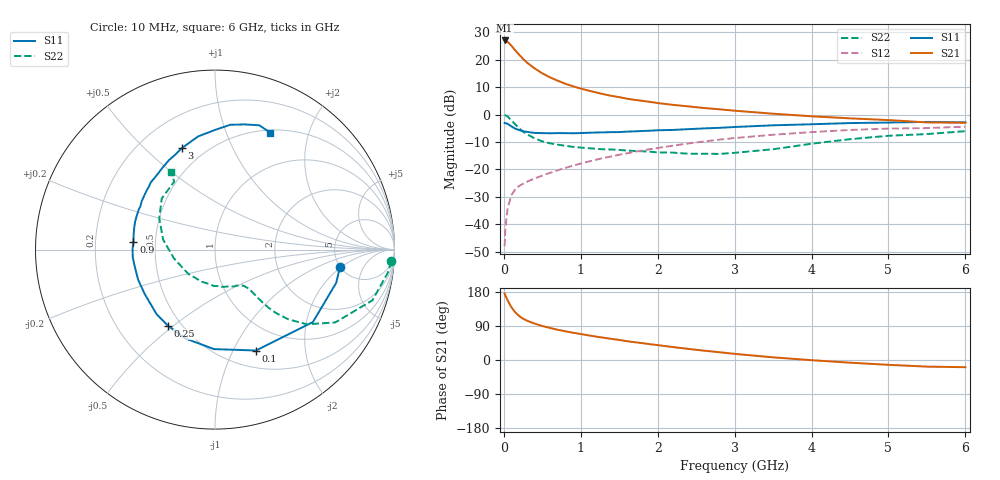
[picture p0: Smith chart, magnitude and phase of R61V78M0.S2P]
! SIEMENS Small Signal Semiconductors
! BFR193
! Si NPN RF Bipolar Junction Transistor in SOT23
! VCE = 1.75 V  IC = 8 mA
! Common Emitter S-Parameters:  May  1996
# GHz  S  MA  R  50
!  f  S11  S21  S12  S22
! GHz  MAG  ANG  MAG  ANG  MAG  ANG  MAG  ANG
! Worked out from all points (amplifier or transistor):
!   36 points, 10 MHz to 6 GHz, reference 50 ohm
!   highest |S21| = 27.0 dB at 10 MHz (marker M1)
!   |S21| within 3 dB of that: start of sweep to 130.2 MHz
!   unconditionally stable (mu >= 1): 771.2 MHz to 1.99 GHz
!   at 250 MHz: K = 0.58, MSG = 22.8 dB, |S12| = -25.2 dB
!   at 1.4 GHz: K = 1.05, MAG = 9.7 dB, |S12| = -15.2 dB
!   at 6 GHz: K = 0.96, MSG = 0.7 dB, |S12| = -4.4 dB
!   S11 on the Smith chart (normalised r, x): 10 MHz: 4.99, -1.88; 100 MHz: 0.69, -1.23; 250 MHz: 0.42, -0.48; 900 MHz: 0.37, +0.04; 3 GHz: 0.37, +0.65; 6 GHz: 0.53, +1.44
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0.01  0.7027 -7.8  22.46 175.3  0.004 88.2  0.9843 -3.8
0.02  0.7004 -15.3  22.03 170.3  0.0085 82.0  0.973 -7.4
0.05  0.6785 -36.5  21.13 157.0  0.0199 72.7  0.9212 -17.9
0.1  0.6068 -67.9  17.96 138.7  0.0345 62.0  0.7833 -31.2
0.15  0.5544 -90.6  14.69 125.3  0.0437 55.9  0.66 -39.1
0.2  0.5219 -108.3  12.32 116.0  0.05 53.0  0.5609 -43.7
0.25  0.4985 -121.7  10.37 109.0  0.055 51.9  0.487 -46.2
0.3  0.4852 -132.1  8.888 103.8  0.0597 52.0  0.438 -47.4
0.4  0.4633 -147.6  6.962 96.1  0.0687 53.1  0.3698 -48.3
0.5  0.4599 -158.6  5.653 89.7  0.0775 55.1  0.3256 -48.6
0.6  0.4568 -167.1  4.778 84.5  0.0867 56.6  0.2994 -48.9
0.7  0.4601 -174.5  4.149 79.8  0.0964 57.9  0.2834 -49.5
0.9  0.457 174.6  3.279 71.9  0.1174 59.4  0.2585 -51.5
1.1  0.4666 164.7  2.74 65.0  0.1394 60.3  0.2447 -55.3
1.3  0.4745 157.0  2.348 58.7  0.1621 60.1  0.2329 -59.5
1.6  0.4898 146.4  1.951 49.7  0.1969 58.7  0.2217 -68.4
2.2  0.5261 128.2  1.503 34.1  0.2719 53.5  0.2028 -91.6
3  0.5943 108.3  1.178 16.2  0.3741 43.0  0.2012 -137.6
3.5  0.6379 98.4  1.038 7.0  0.4293 35.2  0.2338 -167.9
4.5  0.7007 83.0  0.855 -7.1  0.5242 19.7  0.3563 150.7
5.5  0.7351 70.4  0.721 -17.5  0.5671 4.1  0.4418 120.9
6  0.721 64.8  0.71 -19.0  0.6036 -0.6  0.4991 119.7
